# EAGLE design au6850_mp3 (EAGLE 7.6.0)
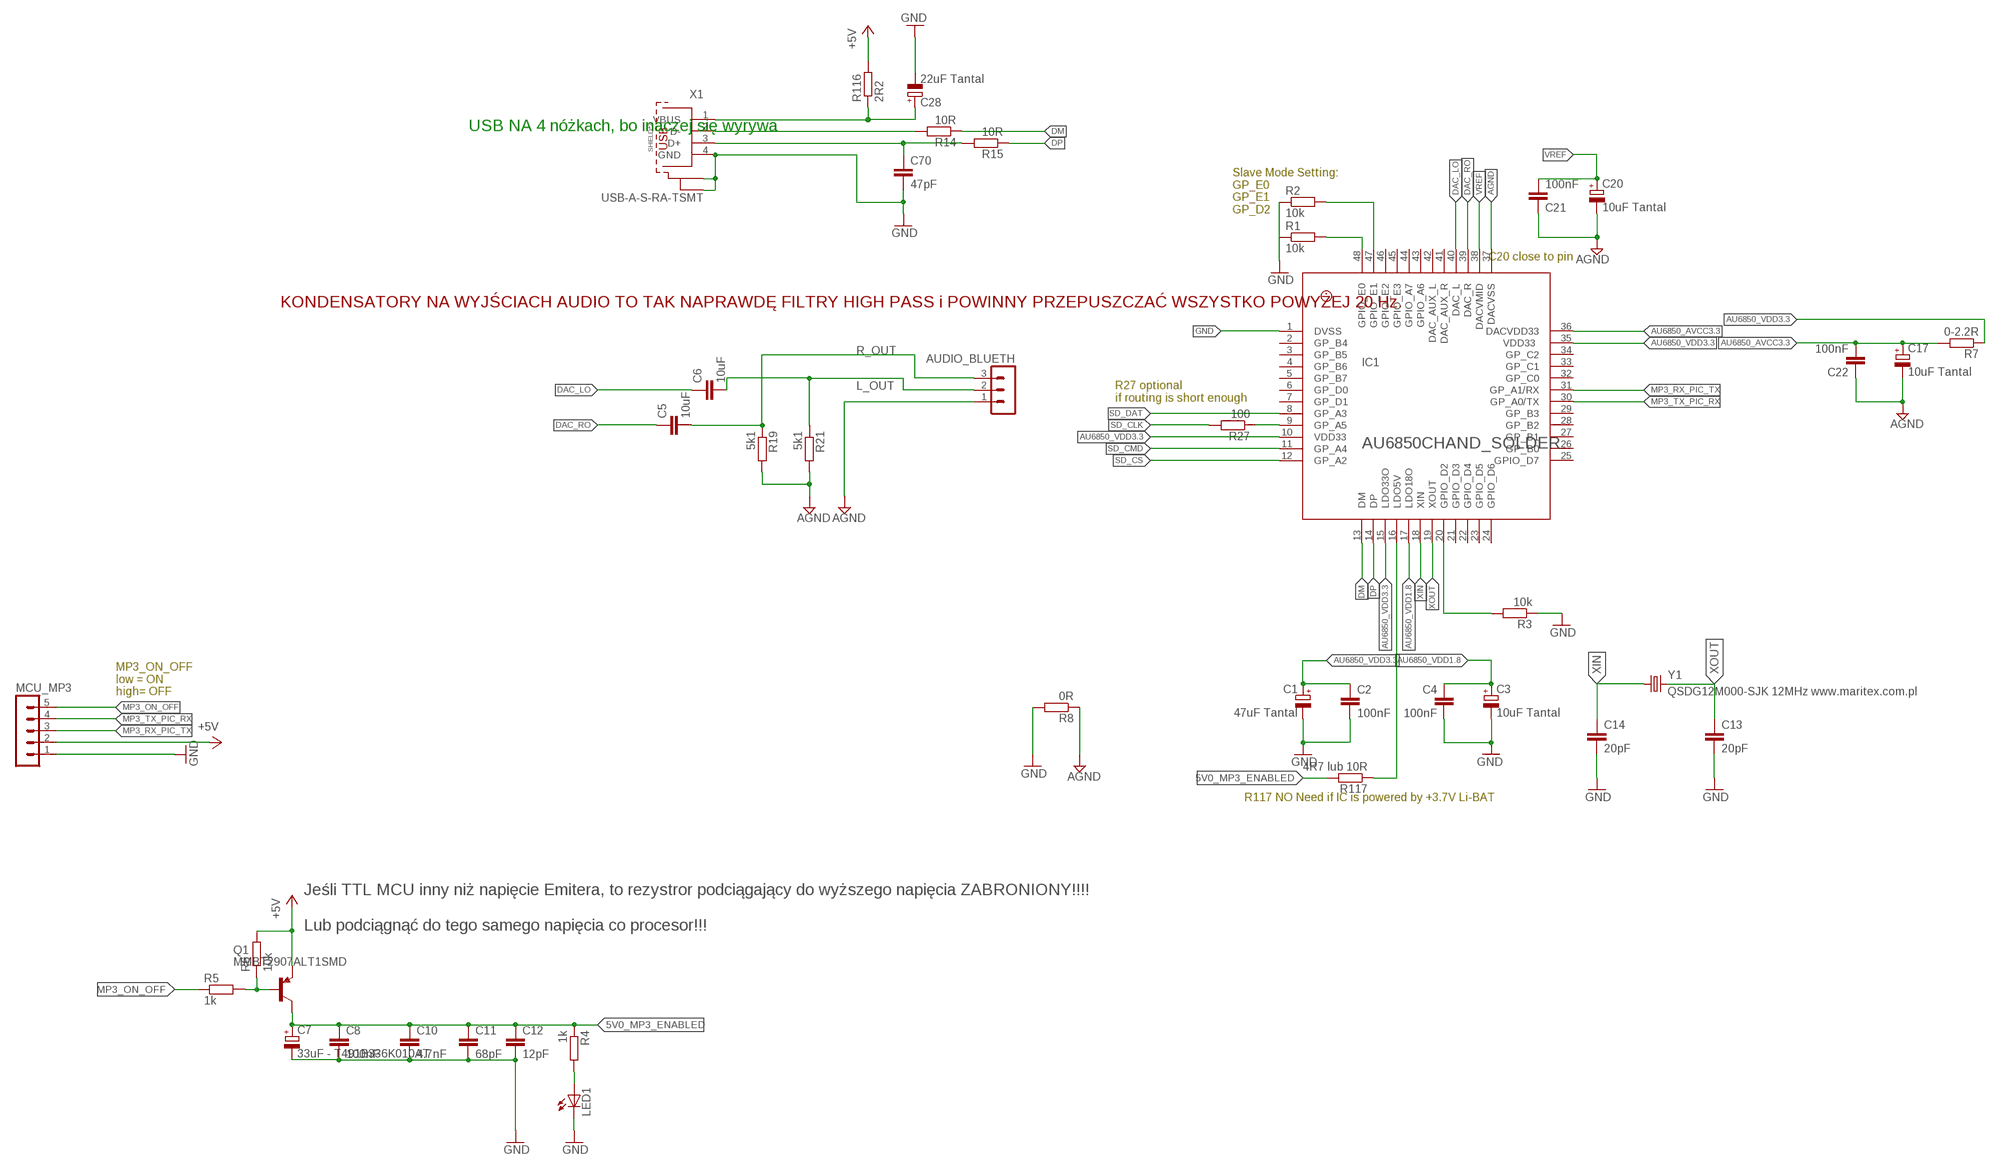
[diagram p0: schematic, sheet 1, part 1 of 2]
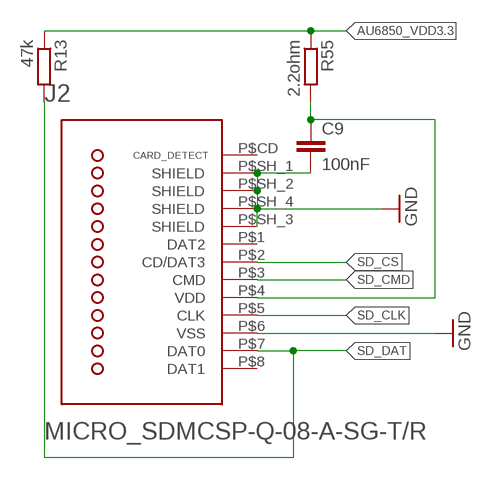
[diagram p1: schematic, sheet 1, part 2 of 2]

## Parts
AUDIO_BLUETH  MA03-1  [MA03-1]
C1  47uF Tantal  CPOL-EUB/3528-21R  [B/3528-21R]
C2  100nF  C-EUC0805  [C0805]
C3  10uF Tantal  CPOL-EUB/3528-21R  [B/3528-21R]
C4  100nF  C-EUC0805  [C0805]
C5  10uF  C-EUC0805  [C0805]
C6  10uF  C-EUC0805  [C0805]
C7  33uF - T491B336K010AT  CPOL-EUSMCB  [SMC_B]
C8  100nF  C-EUC0805  [C0805]
C9  100nF  C-EUC0805  [C0805]
C10  4.7nF  C-EUC0805  [C0805]
C11  68pF  C-EUC0805  [C0805]
C12  12pF  C-EUC0603K  [C0603K]
C13  20pF  C-EUC0805  [C0805]
C14  20pF  C-EUC0805  [C0805]
C17  10uF Tantal  CPOL-EUB/3528-21R  [B/3528-21R]
C20  10uF Tantal  CPOL-EUB/3528-21R  [B/3528-21R]
C21  100nF  C-EUC0805  [C0805]
C22  100nF  C-EUC0805  [C0805]
C28  22uF Tantal  CPOL-EUSMCB  [SMC_B]
C70  47pF  C-EUC0805  [C0805]
IC1  AU6850CHAND_SOLDER  [LQFP48-7X7_3MM]
J2  MICRO_SDMCSP-Q-08-A-SG-T/R  [MICRO_SD_8PINS]
LED1  LED3MM  [LED3MM]
MCU_MP3  MA05-1  [MA05-1]
Q1  MMBT2907ALT1SMD  [SOT23-BEC]
R1  10k  R-EU_R0805  [R0805]
R2  10k  R-EU_R0805  [R0805]
R3  10k  R-EU_R0805  [R0805]
R4  1k  R-EU_M0805  [M0805]
R5  1k  R-EU_M0805  [M0805]
R6  10k  R-EU_M0805  [M0805]
R7  0-2.2R  R-EU_R0805  [R0805]
R8  0R  R-EU_R0805  [R0805]
R13  47k  R-EU_R0805  [R0805]
R14  10R  R-EU_R0805  [R0805]
R15  10R  R-EU_R0805  [R0805]
R19  5k1  R-EU_R0805  [R0805]
R21  5k1  R-EU_R0805  [R0805]
R27  100  R-EU_R0805  [R0805]
R55  2.2ohm  R-EU_R0805  [R0805]
R116  2R2  R-EU_R0805  [R0805]
R117  4R7 lub 10R  R-EU_R0805  [R0805]
X1  USB-A-S-RA-TSMT  [USB-A-S-RA-TSMT]
Y1  QSDG12M000-SJK 12MHz www.maritex.com.pl  CRYSTALSMD  [HC49UP]

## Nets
5V0_MP3_ENABLED: C7.+ C8.1 C10.1 C11.1 C12.1 Q1.C R4.1 R117.2
+5V: MCU_MP3.2 Q1.E R6.2 R116.2
AGND: AUDIO_BLUETH.1 C17.- C20.- C21.1 C22.1 IC1.37(DACVSS) R8.1 R19.2 R21.2
AU6850_AVCC3.3: C17.+ C22.2 IC1.36(DACVDD33) R7.2
AU6850_VDD1.8: C3.+ C4.1 IC1.17(LDO18O)
AU6850_VDD3.3: C1.+ C2.1 IC1.10(VDD33) IC1.15(LDO33O) IC1.35(VDD33) R7.1 R13.1 R55.1
DAC_LO: C6.1 IC1.40(DAC_L)
DAC_RO: C5.1 IC1.39(DAC_R)
DM: IC1.13(DM) R14.1
DP: IC1.14(DP) R15.1
GND: C1.- C2.2 C3.- C4.2 C7.- C8.2 C9.2 C10.2 C11.2 C12.2 C13.2 C14.2 C28.- C70.2 IC1.1(DVSS) J2.P$6(VSS) J2.P$SH_1(1_GND_PAD) J2.P$SH_2(2_GND_PAD) J2.P$SH_3(3_GND_PAD) J2.P$SH_4(4_GND_PAD) LED1.K(C) MCU_MP3.1 R1.1 R2.1 R3.1 R8.2 X1.4(GND) X1.5(SH1) X1.6(SH2)
L_OUT: AUDIO_BLUETH.2 C6.2 R21.1
MP3_ON_OFF: MCU_MP3.5 R5.1
MP3_RX_PIC_TX: IC1.31(GP_A1/RX) MCU_MP3.3
MP3_TX_PIC_RX: IC1.30(GP_A0/TX) MCU_MP3.4
N$1: LED1.A R4.2
N$2: Q1.B R5.2 R6.1
N$4: IC1.16(LDO5V) R117.1
N$5: IC1.9(GP_A5) R27.1
N$8: C28.+ R116.1 X1.1(VBUS)
N$9: C70.1 R15.2 X1.3(D+)
N$10: R14.2 X1.2(D-)
N$14: C9.1 J2.P$4(VDD) R55.2
R_OUT: AUDIO_BLUETH.3 C5.2 R19.1
SD_CLK: J2.P$5(CLK) R27.2
SD_CMD: IC1.11(GP_A4) J2.P$3(CMD)
SD_CS: IC1.12(GP_A2) J2.P$2(CD/DAT3)
SD_DAT: IC1.8(GP_A3) J2.P$7(DAT0) R13.2
SLAVE_D2: IC1.20(GPIO_D2) R3.2
SLAVE_E0: IC1.48(GPIO_E0) R1.2
SLAVE_E1: IC1.47(GPIO_E1) R2.2
VREF: C20.+ C21.2 IC1.38(DACVMID)
XIN: C14.1 IC1.18(XIN) Y1.1
XOUT: C13.1 IC1.19(XOUT) Y1.2
Unconnected: IC1.2(GP_B4) IC1.3(GP_B5) IC1.4(GP_B6) IC1.5(GP_B7) IC1.6(GP_D0) IC1.7(GP_D1) IC1.21(GPIO_D3) IC1.22(GPIO_D4) IC1.23(GPIO_D5) IC1.24(GPIO_D6) IC1.25(GPIO_D7) IC1.26(GP_B0) IC1.27(GP_B1) IC1.28(GP_B2) IC1.29(GP_B3) IC1.32(GP_C0) IC1.33(GP_C1) IC1.34(GP_C2) IC1.41(DAC_AUX_R) IC1.42(DAC_AUX_L) IC1.43(GPIO_A6) IC1.44(GPIO_A7) IC1.45(GPIO_E3) IC1.46(GPIO_E2) J2.P$1(DAT2) J2.P$8(DAT1) J2.P$CD(CARD_DETECT_SW)

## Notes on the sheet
- USB NA 4 nóżkach, bo inaczej się wyrywa
- Slave Mode Setting:
  GP_E0
  GP_E1
  GP_D2
- C20 close to pin
- KONDENSATORY NA WYJŚCIACH AUDIO TO TAK NAPRAWDĘ FILTRY HIGH PASS i POWINNY PRZEPUSZCZAĆ WSZYSTKO POWYŻEJ 20 Hz.
- R27 optional
  if routing is short enough
- MP3_ON_OFF
  low = ON
  high= OFF
- R117 NO Need if IC is powered by +3.7V Li-BAT
- Jeśli TTL MCU inny niż napięcie Emitera, to rezystror podciągający do wyższego napięcia ZABRONIONY!!!!
  
  Lub podciągnąć do tego samego napięcia co procesor!!!

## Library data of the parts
AUDIO_BLUETH = con-lstb:MA03-1: PIN HEADER; OC_FARNELL: unknown; OC_NEWARK: unknown
C1 = rcl:CPOL-EU: POLARIZED CAPACITOR, European symbol; PARTNUM: TAJB476K010R; SUPPLIER: TME
C2 C4-C6 C21 C22 = rcl:C-EU: CAPACITOR, European symbol
C3 = rcl:CPOL-EU: POLARIZED CAPACITOR, European symbol; PARTNUM: TAJA106K010R; SUPPLIER: TME
C7 = resistor:CPOL-EU: POLARIZED CAPACITOR, European symbol; PARTNUM: TAJB336K010R; SUPPLIER: TME
C8-C14 C70 = resistor:C-EU: CAPACITOR, European symbol
C17 C20 = rcl:CPOL-EU: POLARIZED CAPACITOR, European symbol
C28 = rcl:CPOL-EU: POLARIZED CAPACITOR, European symbol; PARTNUM: TAJB226M010R; SUPPLIER: TME
IC1 = mvsilicon:AU6850C
J2 = ADAM_TECH_SD_Card:MICRO_SD: Adam Tech; PARTNUM: MCSP-Q-08-A-SG-T/R; SUPPLIER: TME
LED1 = led:LED: LED
MCU_MP3 = con-lstb:MA05-1: PIN HEADER; OC_FARNELL: unknown; OC_NEWARK: unknown
Q1 = transistor-pnp:MMBT2907*: PNP Transistror
R1-R8 R13-R15 R19 R21 R27 R55 R116 R117 = rcl:R-EU_: RESISTOR, European symbol
X1 = ADAM_TECH_USB-A-S-RA-TSMT:USB-A-S-RA-TSMT: MULTICOMP - USB-A-S-RA-TSMT - USB, 3.0 TYPE A, RECEPTACLE, SMT CUI -UJ2-AH-1-SMT-TR, 3.0 TYPE A, RECEPTACLE, SMT AdamTech - USB-A-S-RA-TSMT - USB, 3.0 TYPE A, RECEPTACLE, SMT Source: Datasheet; DESCRIPTION: MULTICOMP - USB-A-S-RA-TSMT - USB, 3.0 TYPE A, RECEPTACLE, SMT; HEIGHT: mm; MANUFACTURER_NAME: MULTICOMP; MANUFACTURER_PART_NUMBER: USB-A-S-RA-TSMT
Y1 = SparkFun-FreqCtrl:CRYSTAL: Various standard crystals. Proven footprints. Spark Fun Electronics SKU : COM-00534; PARTNUM: 12.00M-SMDHC49S; SUPPLIER: TME

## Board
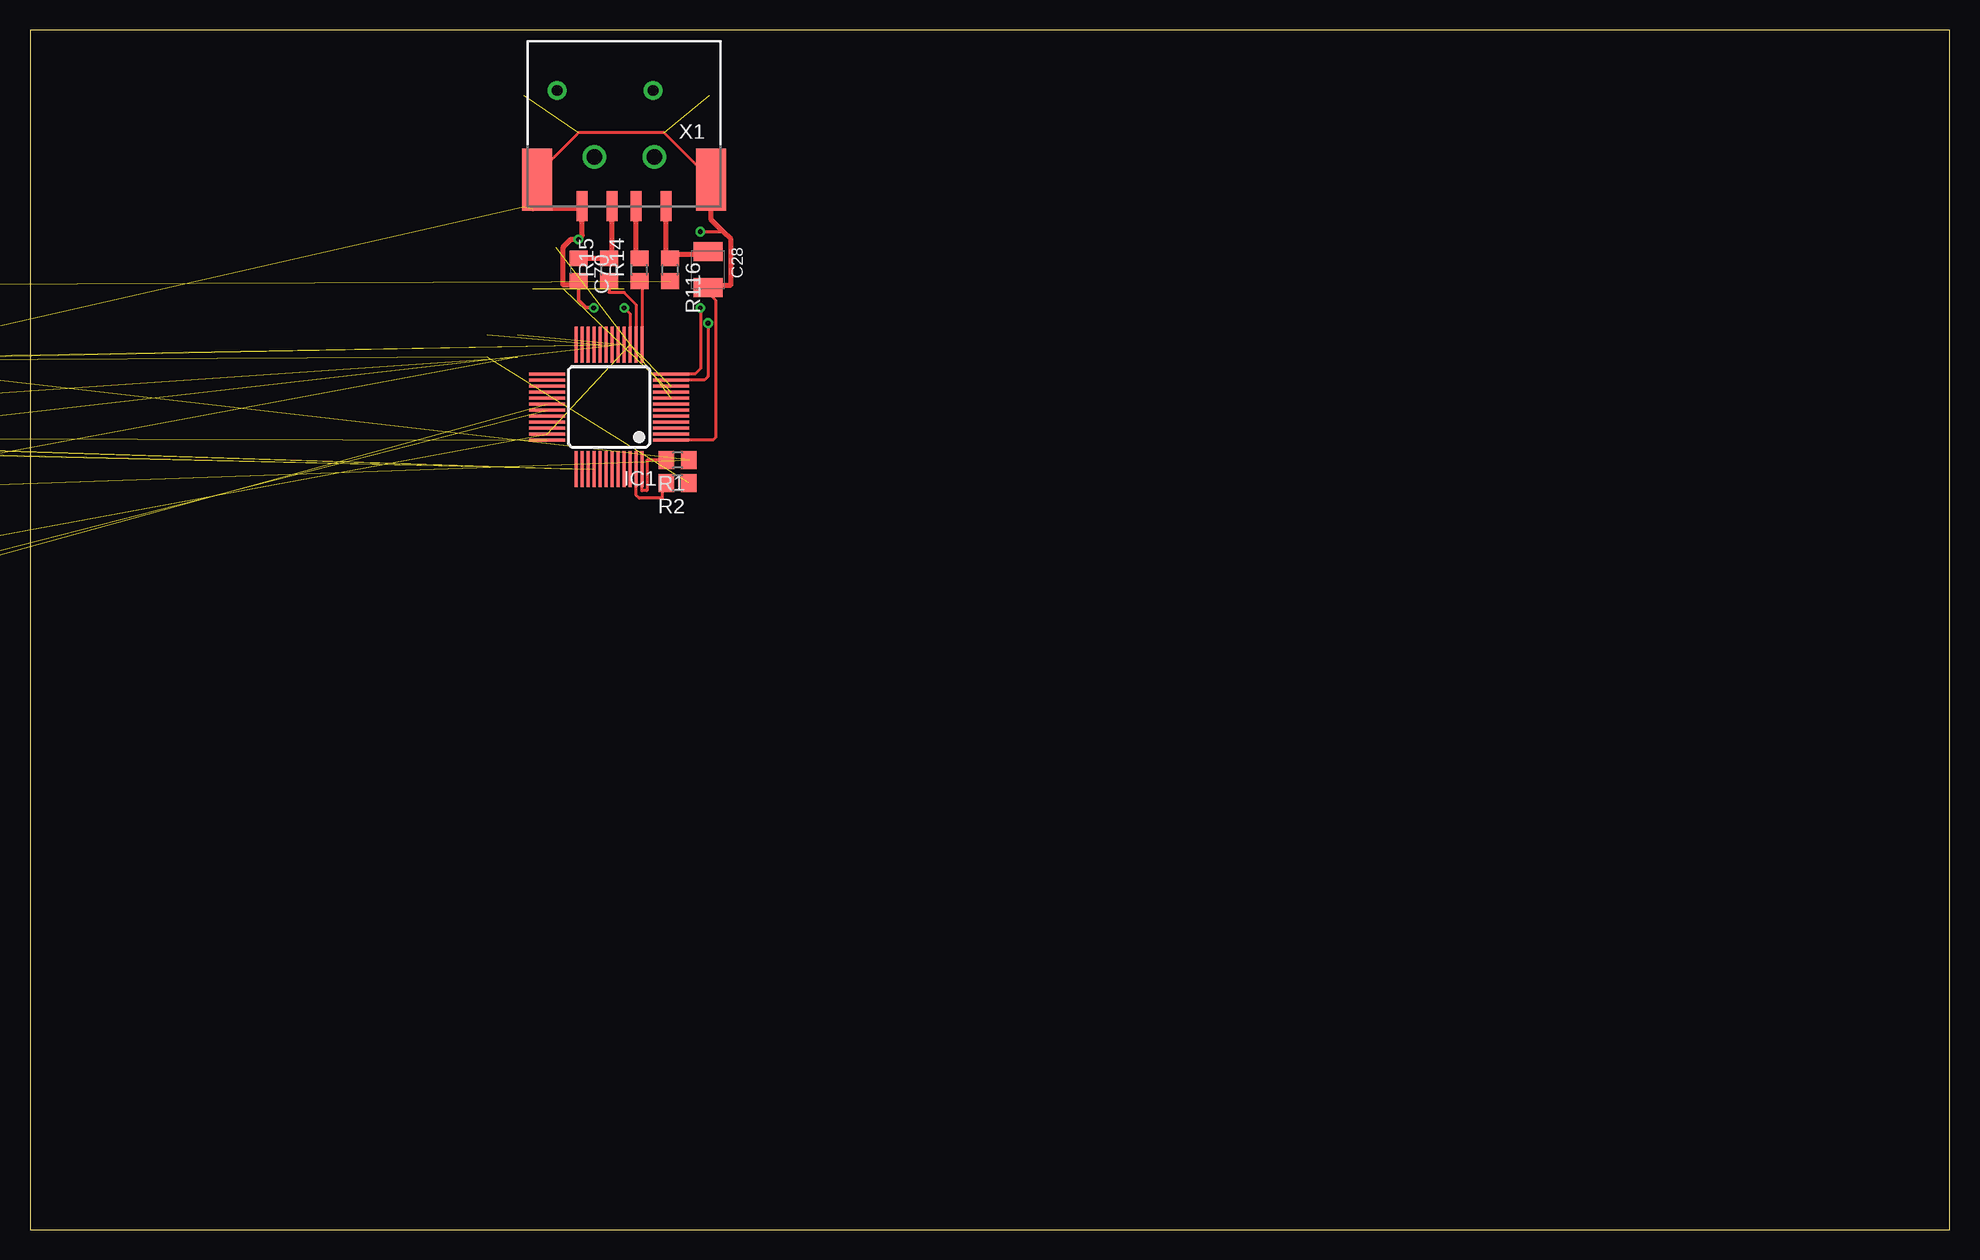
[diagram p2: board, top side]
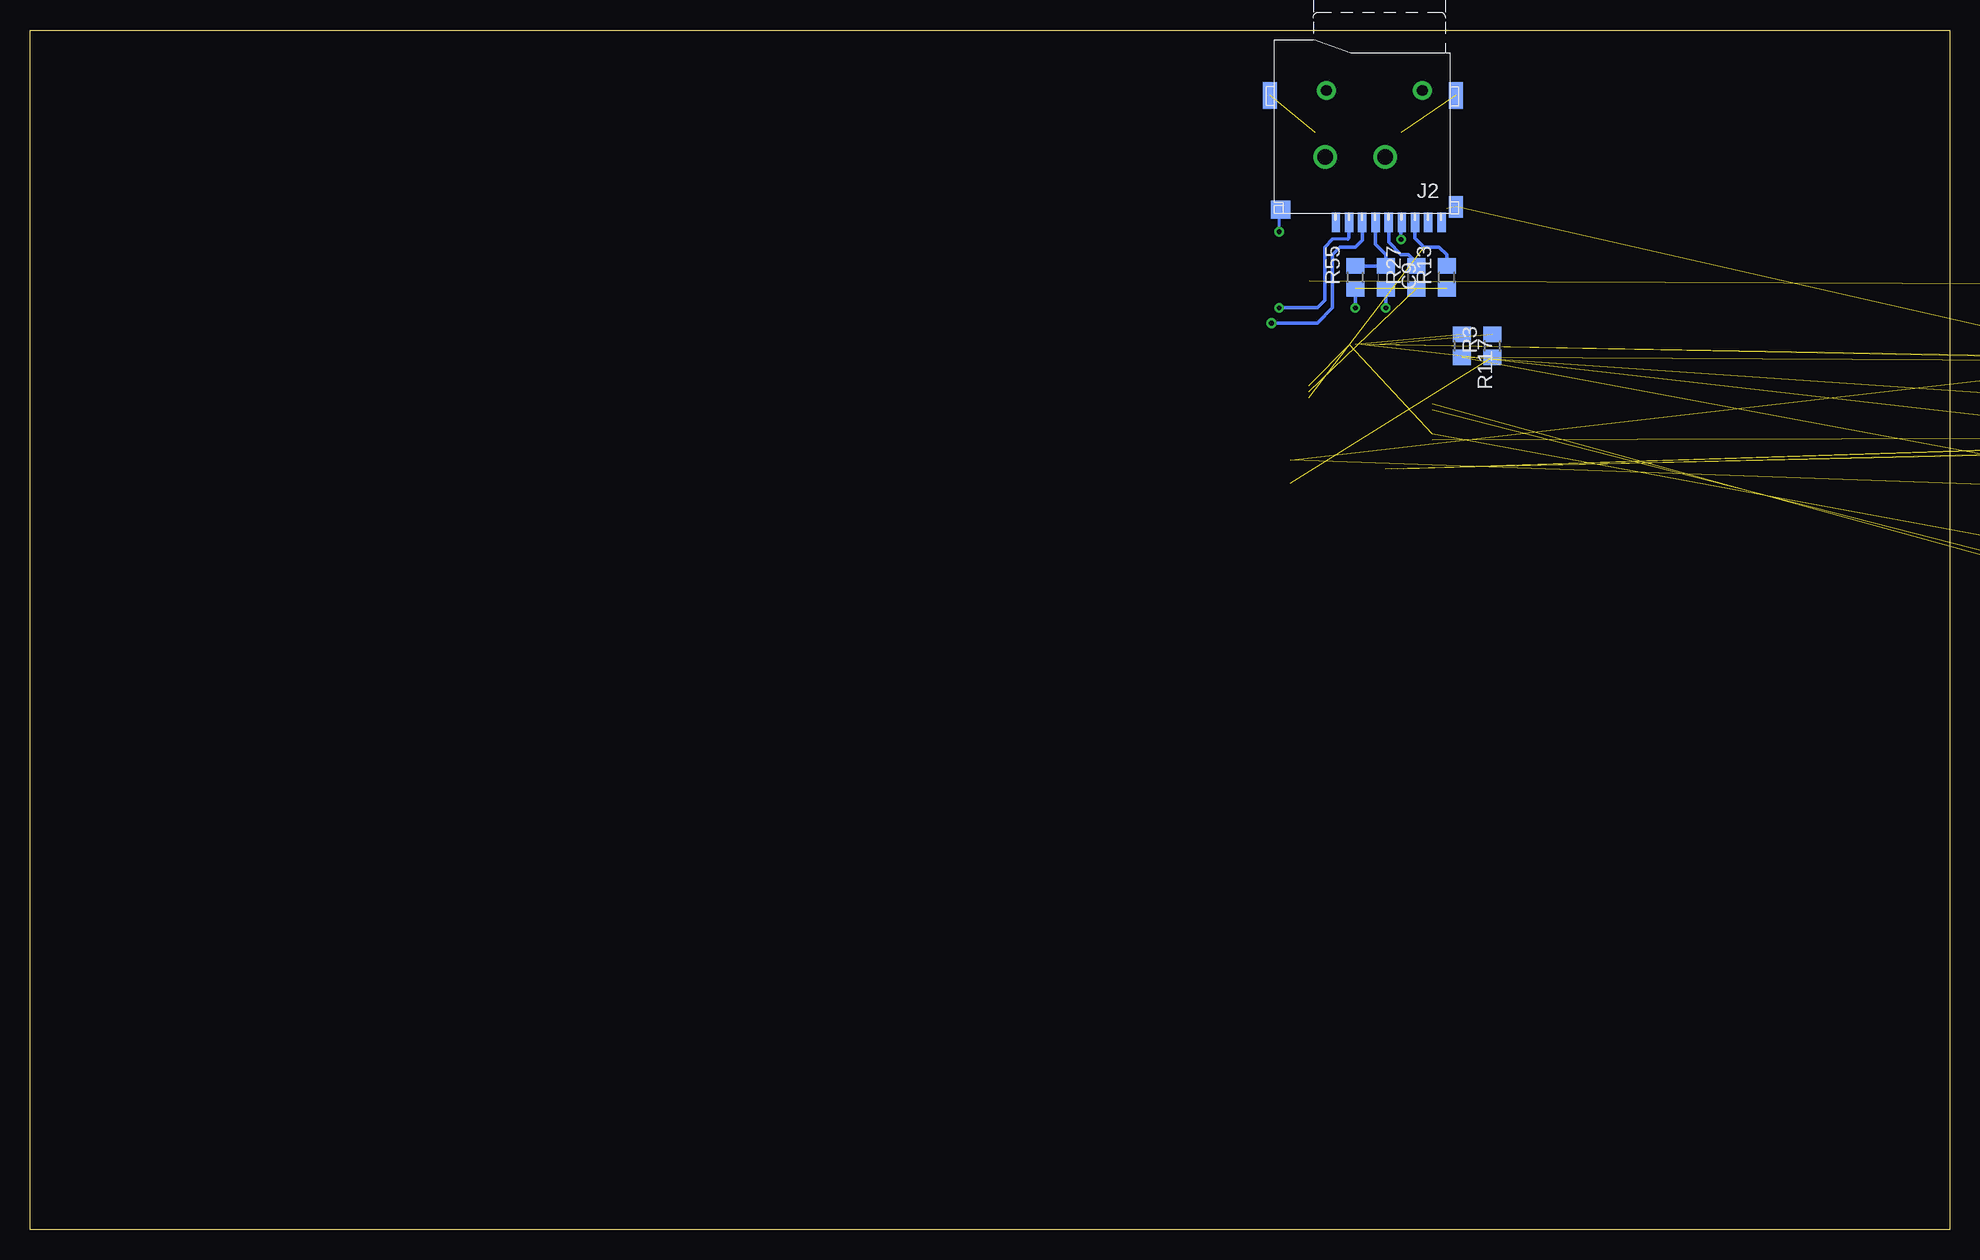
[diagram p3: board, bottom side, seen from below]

Size 160 x 100 mm. Coordinates in mm from the lower left corner, seen from the top.
Outline: 0,0 160,0 160,100 0,100 0,0
Copper layers (1*16): Top 0.035mm / dielectric 1.5mm / Bottom 0.035mm
Design rules "default": minimum track width 10mil, minimum drill 24mil, track to track 8mil, track to pad 8mil, pad to pad 8mil, via to via 8mil, smd to smd 8mil, copper to edge 40mil, drill to drill 8mil, minimum pad ring 10mil, minimum via ring 8mil, stop-mask expansion 4mil, vias tented up to drill 0mil, thermal gap 10mil

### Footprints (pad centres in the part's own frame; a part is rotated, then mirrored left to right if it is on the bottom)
MA03-1 = drill 1.016 long: 1 -2.54,0; 2 0,0; 3 2.54,0
B/3528-21R = smd 1.95 x 2.5: + 1.525,0; - -1.525,0
C0805 = smd 1.3 x 1.5: 1 -0.95,0; 2 0.95,0
SMC_B = smd 1.6 x 2.4: + -1.5,0; - 1.5,0
C0603K = smd 1.05 x 1.08: 1 -0.875,0; 2 0.875,0
LQFP48-7X7_3MM = smd 3 x 0.254: 1 -5.175,2.75; 2 -5.175,2.25; 3 -5.175,1.75; 4 -5.175,1.25; 5 -5.175,0.75; 6 -5.175,0.25; 7 -5.175,-0.25; 8 -5.175,-0.75; 9 -5.175,-1.25; 10 -5.175,-1.75; 11 -5.175,-2.25; 12 -5.175,-2.75; 25 5.175,-2.75; 26 5.175,-2.25; 27 5.175,-1.75; 28 5.175,-1.25; 29 5.175,-0.75; 30 5.175,-0.25; 31 5.175,0.25; 32 5.175,0.75; 33 5.175,1.25; 34 5.175,1.75; 35 5.175,2.25; 36 5.175,2.75 | smd 0.254 x 3: 13 -2.75,-5.175; 14 -2.25,-5.175; 15 -1.75,-5.175; 16 -1.25,-5.175; 17 -0.75,-5.175; 18 -0.25,-5.175; 19 0.25,-5.175; 20 0.75,-5.175; 21 1.25,-5.175; 22 1.75,-5.175; 23 2.25,-5.175; 24 2.75,-5.175; 37 2.75,5.175; 38 2.25,5.175; 39 1.75,5.175; 40 1.25,5.175; 41 0.75,5.175; 42 0.25,5.175; 43 -0.25,5.175; 44 -0.75,5.175; 45 -1.25,5.175; 46 -1.75,5.175; 47 -2.25,5.175; 48 -2.75,5.175
MICRO_SD_8PINS = drill 0.9 pad 1.575: 1 -4.95,-10.5; 15 3.05,-10.5 | smd 0.7 x 1.6: P$1 2.25,0.5; P$2 1.15,0.5; P$3 0.05,0.5; P$4 -1.05,0.5; P$5 -2.15,0.5; P$6 -3.25,0.5; P$7 -4.35,0.5; P$8 -5.45,0.5; P$CD -6.55,0.5 | smd 1.2 x 2.2: P$SH_1 -7.75,-10.1; P$SH_2 7.75,-10.1 | smd 1.2 x 1.8: P$SH_3 -7.75,-0.8 | smd 1.6 x 1.5: P$SH_4 6.85,-0.55
LED3MM = drill 0.813 octagon: A -1.27,0; K 1.27,0
MA05-1 = drill 1.016 long: 1 -5.08,0; 2 -2.54,0; 3 0,0; 4 2.54,0; 5 5.08,0
SOT23-BEC = smd 1 x 1.4: B -0.95,-1.1; C 0,1.1; E 0.95,-1.1
R0805 = smd 1.3 x 1.5: 1 -0.95,0; 2 0.95,0
M0805 = smd 1.3 x 1.6: 1 -0.95,0; 2 0.95,0
USB-A-S-RA-TSMT = smd 0.9 x 2.5: 1 -3.5,13.75; 2 -1,13.75; 3 1,13.75; 4 3.5,13.75 | smd 2.5 x 5.15: 5 -7.25,11.55; 6 7.25,11.55 | drill 1.3 pad 1.95: 7 -2.5,9.65; 8 2.5,9.65
HC49UP = smd 5.334 x 1.93: 1 -4.826,0; 2 4.826,0

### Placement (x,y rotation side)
AUDIO_BLUETH  not placed on the board
C1  not placed on the board
C2  not placed on the board
C3  not placed on the board
C4  not placed on the board
C5  not placed on the board
C6  not placed on the board
C7  not placed on the board
C8  not placed on the board
C9  46.99,79.38 270 bottom
C10  not placed on the board
C11  not placed on the board
C12  not placed on the board
C13  not placed on the board
C14  not placed on the board
C17  not placed on the board
C20  not placed on the board
C21  not placed on the board
C22  not placed on the board
C28  56.52,80.01 270 top
C70  45.72,80.01 270 top
IC1  48.26,68.58 180 top
J2  48.9,84.45 180 bottom
LED1  not placed on the board
MCU_MP3  not placed on the board
Q1  not placed on the board
R1  53.98,64.14 180 top
R2  53.98,62.23 180 top
R3  38.1,73.66 90 bottom
R4  not placed on the board
R5  not placed on the board
R6  not placed on the board
R7  not placed on the board
R8  not placed on the board
R13  41.91,79.38 90 bottom
R14  50.8,80.01 90 top
R15  48.26,80.01 90 top
R19  not placed on the board
R21  not placed on the board
R27  44.45,79.38 90 bottom
R55  49.53,79.38 90 bottom
R116  53.34,80.01 270 top
R117  40.64,73.66 270 bottom
X1  49.53,99.06 180 top
Y1  not placed on the board

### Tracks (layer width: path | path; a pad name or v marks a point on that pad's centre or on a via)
5V0_MP3_ENABLED  (7 unrouted)
+5V  (3 unrouted)
AGND  (8 unrouted)
AU6850_AVCC3.3  (3 unrouted)
AU6850_VDD1.8  (2 unrouted)
AU6850_VDD3.3  (via drill 0.4)  (6 unrouted)
  Top 0.254: v49.53,76.83 50.01,76.36 IC1.15
  Bottom 0.305: R55.1 v49.53,76.83
DAC_LO  (1 unrouted)
DAC_RO  (1 unrouted)
DM
  Top 0.254: R14.1 51.01,79.06 IC1.13
DP
  Top 0.254: R15.1 48.26,78.11 49.53,78.11 50.51,77.12 IC1.14
GND  (via drill 0.4)  (20 unrouted)
  Top 0.254: IC1.1 56.94,65.83 57.15,66.04 57.15,77.47 56.52,78.11 C28.- | v55.88,83.19 57.78,83.19 | X1.5 52.85,91.44 45.72,91.44 42.28,88 X1.6
  Top 0.305: C70.2 45.72,77.47 46.35,76.83 v46.99,76.83
  Top 0.406: C70.2 45.4,78.74 44.45,78.74 44.45,81.92 45.09,82.55 v45.72,82.55 46.03,82.86 X1.4 45.81,85.09 41.91,85.09 42.28,85.46 X1.6 | C28.- 56.74,78.74 58.42,78.74 58.42,82.55 57.78,83.19 56.78,84.19 X1.5
  Bottom 0.254: J2.P$SH_4 55.88,84.87 v55.88,83.19
  Bottom 0.305: J2.P$6 45.72,83.88 v45.72,82.55 | C9.2 v46.99,76.83
L_OUT  (2 unrouted)
MP3_ON_OFF  (1 unrouted)
MP3_RX_PIC_TX  (1 unrouted)
MP3_TX_PIC_RX  (1 unrouted)
N$1  (1 unrouted)
N$2  (2 unrouted)
N$4  (1 unrouted)
N$5  (1 unrouted)
N$8
  Top 0.406: X1.1 53.03,81.27 R116.1 53.34,81.28 56.28,81.28 C28.+
N$9
  Top 0.406: X1.3 48.53,81.23 R15.2 C70.1
N$10
  Top 0.406: R14.2 50.53,81.23 X1.2
N$14
  Bottom 0.305: R55.2 C9.1 46.99,81.28 47.84,82.14 J2.P$4
R_OUT  (2 unrouted)
SD_CLK
  Bottom 0.305: J2.P$5 46.74,82.31 45.72,81.28 45.09,81.28 44.45,80.64 R27.2
SD_CMD  (via drill 0.4)
  Top 0.254: v56.52,75.56 56.52,71.12 56.23,70.83 IC1.11
  Bottom 0.305: J2.P$3 48.95,82.5 49.53,81.92 50.8,81.92 51.44,81.28 51.44,76.83 52.7,75.56 v56.52,75.56
SD_CS  (via drill 0.4)
  Top 0.254: v55.88,76.83 55.88,71.75 55.45,71.33 IC1.12
  Bottom 0.254: 50.16,82.55 51.44,82.55
  Bottom 0.305: J2.P$2 50.05,82.67 50.16,82.55 | 51.44,82.55 52.07,81.92 52.07,77.47 52.7,76.83 v55.88,76.83
SD_DAT  (1 unrouted)
  Bottom 0.305: R13.2 41.91,81.28 42.55,81.92 43.81,81.92 44.55,82.64 J2.P$7
SLAVE_D2  (1 unrouted)
SLAVE_E0
  Top 0.254: R1.2 51.44,64.14 51.44,61.59 51.01,61.59 IC1.48
SLAVE_E1
  Top 0.254: R2.2 52.7,62.23 52.7,60.96 50.8,60.96 50.51,61.25 IC1.47
VREF  (2 unrouted)
XIN  (2 unrouted)
XOUT  (2 unrouted)

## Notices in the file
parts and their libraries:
SparkFun-FreqCtrl: Licensing: Creative Commons ShareAlike 4.0 International - https://creativecommons.org/licenses/by-sa/4.0
